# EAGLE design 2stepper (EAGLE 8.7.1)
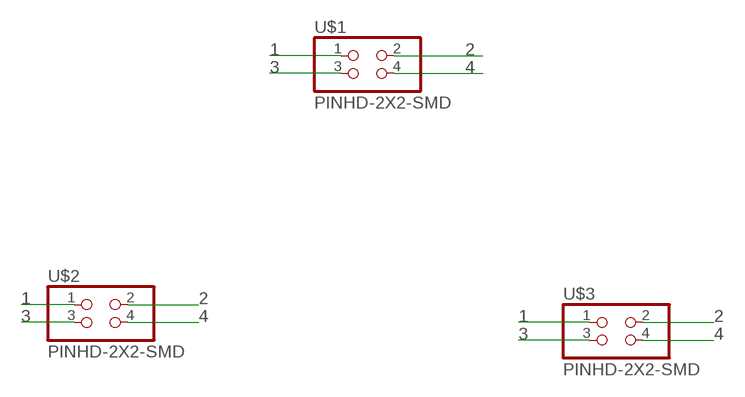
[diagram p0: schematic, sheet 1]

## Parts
U$1  PINHD-2X2-SMD  [2X02SMD]
U$2  PINHD-2X2-SMD  [2X02SMD]
U$3  PINHD-2X2-SMD  [2X02SMD]

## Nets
1: U$1.1 U$2.1 U$3.1
2: U$1.2 U$2.2 U$3.2
3: U$1.3 U$2.3 U$3.3
4: U$1.4 U$2.4 U$3.4

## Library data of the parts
U$1-U$3 = fab:PINHD-2X2-SMD

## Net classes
0 default: width 0.66 mm, clearance 0.4 mm

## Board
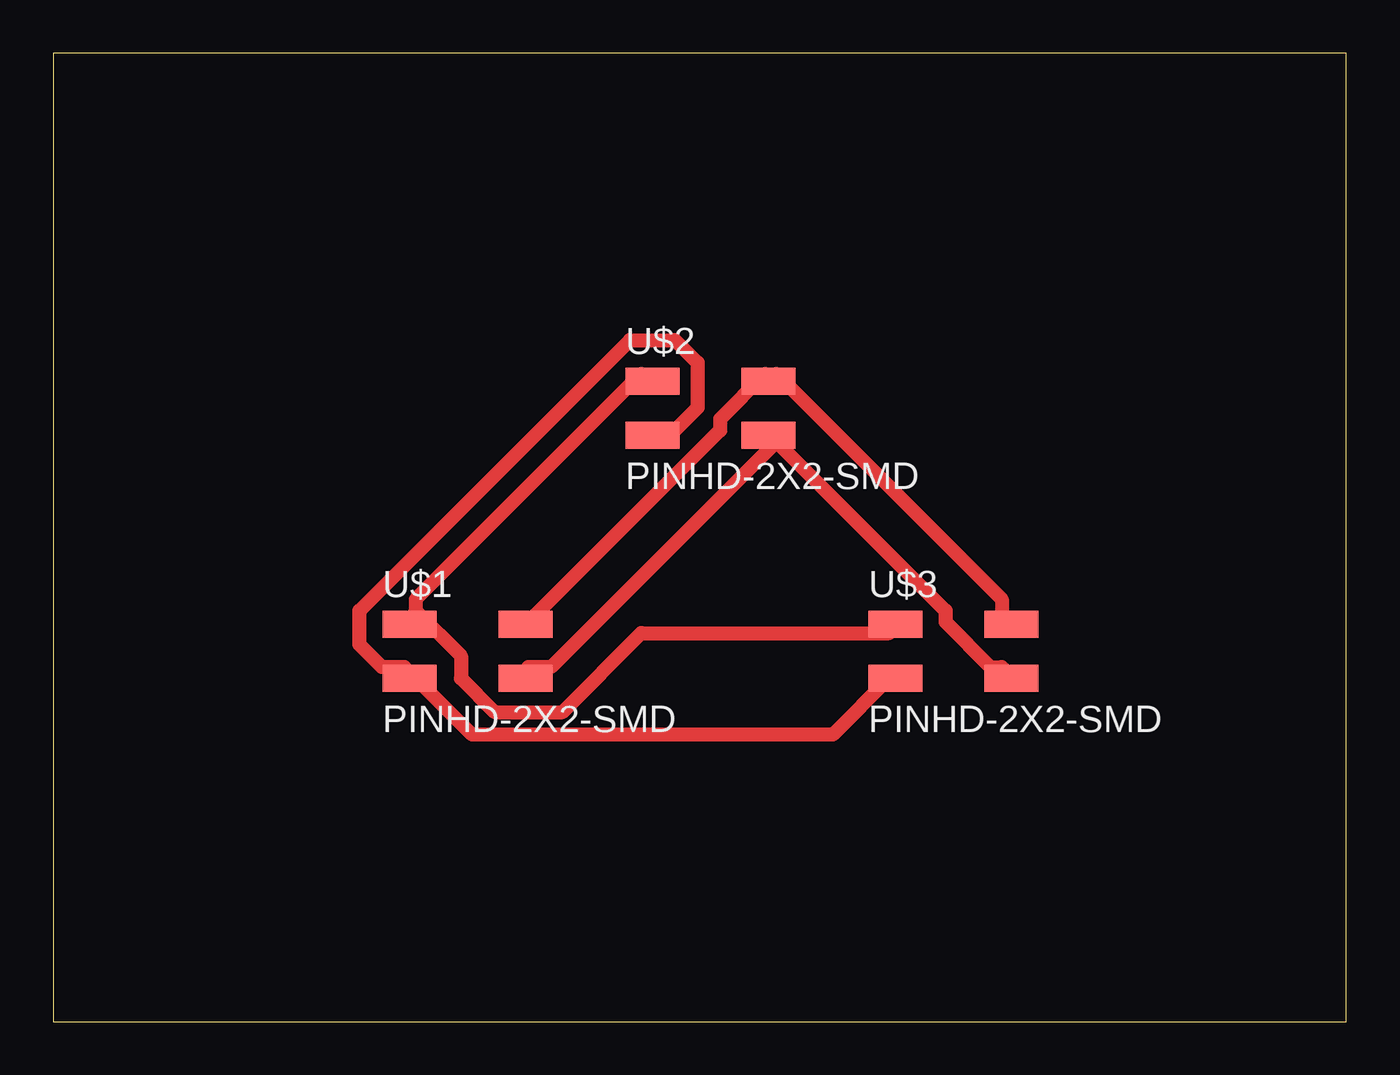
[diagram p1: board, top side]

Size 60.84 x 45.54 mm. Coordinates in mm from the lower left corner, seen from the top.
Outline: 0,0 60.84,0 60.84,45.54 0,45.54 0,0
Copper layers (1*16): Top 0.035mm / dielectric 1.5mm / Bottom 0.035mm
Design rules "default": minimum track width 6mil, minimum drill 0.35mm, track to track 6mil, track to pad 6mil, pad to pad 6mil, via to via 6mil, smd to smd 6mil, copper to edge 40mil, drill to drill 6mil, minimum pad ring 10mil, minimum via ring 8mil, stop-mask expansion 4mil, vias tented up to drill 0mil, thermal gap 10mil

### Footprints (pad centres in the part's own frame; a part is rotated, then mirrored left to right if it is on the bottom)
2X02SMD = smd 2.54 x 1.27: 1 -2.54,1.27; 2 2.92,1.27; 3 -2.54,-1.27; 4 2.92,-1.27

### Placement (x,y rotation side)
U$1  19.3,17.42 0 top
U$2  30.73,28.85 0 top
U$3  42.16,17.42 0 top

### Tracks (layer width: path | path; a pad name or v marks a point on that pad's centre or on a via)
1
  Top 0.66: 17.06,19.32 17.06,19.85 27.66,30.46 U$2.1 | 17.06,19.32 17.06,18.79 U$1.1 17.06,19.32 | 17.06,19.32 19.18,17.2 19.18,16.14 20.77,14.55 23.95,14.55 27.66,18.26 39.33,18.26 U$3.1
2
  Top 0.66: U$1.2 22.36,18.79 31.38,27.81 31.38,28.34 33.5,30.46 U$2.2 34.03,30.46 44.63,19.85 44.63,18.79 U$3.2
3
  Top 0.66: U$3.3 39.33,16.14 36.68,13.49 19.71,13.49 17.06,16.14 U$1.3 16.53,16.67 15.47,16.67 14.41,17.73 14.41,19.32 27.13,32.05 29.25,32.05 30.32,30.99 30.32,28.87 29.25,27.81 28.2,27.81 U$2.3
4
  Top 0.66: 34.03,27.28 23.42,16.67 22.36,16.67 U$1.4 | 34.03,27.28 41.98,19.32 41.98,18.79 44.1,16.67 44.63,16.67 U$3.4 | 34.03,27.28 U$2.4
